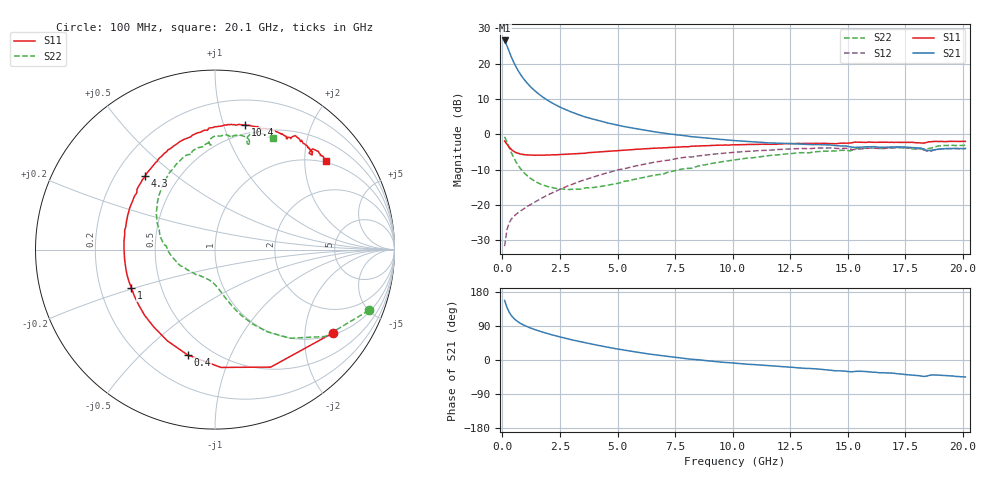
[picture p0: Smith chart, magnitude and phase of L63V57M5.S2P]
!  Infineon Technologies AG
! BFR380L3 , PF131585-7, No.6, Th 09.10.01, soldered on pcb-board, measured with PP GSG850
!  Vce=3.5 V,  Ic=7.5 mA
! Common Emitter S-Parameters:  15. November 2001
#  GHz  S  MA  R  50
! f  S11  S21  S12  S22
! GHz  Mag  Ang  Mag  Ang  Mag  Ang  Mag  Ang
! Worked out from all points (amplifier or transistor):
!   201 points, 100 MHz to 20.1 GHz, reference 50 ohm
!   highest |S21| = 26.5 dB at 100 MHz (marker M1)
!   |S21| within 3 dB of that: start of sweep to 289.7 MHz
!   unconditionally stable (mu >= 1): 1.99 GHz to 4.519 GHz
!   at 3.4 GHz: K = 1.03, MAG = 8.1 dB, |S12| = -13.2 dB
!   at 10.1 GHz: K = 0.94, MSG = 1.6 dB, |S12| = -5.1 dB
!   at 20.1 GHz: K = 0.99, MSG = 0.0 dB, |S12| = -4.0 dB
!   S11 on the Smith chart (normalised r, x): 100 MHz: 1.06, -2.77; 400 MHz: 0.38, -0.70; 1 GHz: 0.34, -0.20; 4.3 GHz: 0.32, +0.39; 10.4 GHz: 0.42, +1.19; 20.1 GHz: 0.95, +2.54
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0.1  0.8036 -35.4  21.17 157.1  0.02627 72.2  0.9217 -21.6
0.2  0.7246 -64.6  17.82 139.0  0.04466 60.2  0.7822 -38.2
0.3  0.6574 -87.1  14.69 126.2  0.05629 52.9  0.6476 -49.7
0.4  0.6068 -104.5  12.21 116.9  0.0638 48.9  0.5422 -57.6
0.5  0.5735 -117.6  10.35 109.9  0.06928 47.2  0.4639 -63.2
0.6  0.5498 -128.3  8.905 104.5  0.07416 46.6  0.4048 -67.4
0.7  0.5368 -136.8  7.816 100.0  0.07855 46.5  0.3594 -70.8
0.8  0.5257 -143.8  6.941 96.3  0.08289 47.0  0.3246 -73.5
1  0.513 -155.2  5.672 90.1  0.09148 48.2  0.2748 -77.8
1.2  0.51 -163.8  4.79 84.9  0.1006 49.7  0.2416 -81.6
1.4  0.5065 -171.1  4.151 80.5  0.11 51.0  0.2186 -84.9
1.6  0.5062 -177.3  3.663 76.3  0.1196 52.2  0.2023 -88.2
1.9  0.5091 174.9  3.125 70.8  0.135 53.3  0.1857 -93.1
2.6  0.5198 160.1  2.344 59.4  0.1725 54.3  0.1688 -105.8
3.5  0.5385 144.7  1.799 46.7  0.224 52.8  0.17 -122.0
4.3  0.565 133.5  1.52 37.0  0.2702 50.1  0.1838 -139.2
6.8  0.6391 104.7  1.062 12.3  0.4145 35.9  0.2702 177.0
10.1  0.7104 78.3  0.8135 -8.4  0.5572 14.1  0.4359 135.5
10.4  0.715 76.3  0.8016 -9.9  0.5676 12.1  0.4487 132.2
13.5  0.7406 60.2  0.716 -22.9  0.6326 -7.8  0.56 103.2
16.8  0.7683 47.6  0.6584 -34.0  0.6373 -24.5  0.6471 79.7
20.1  0.7942 38.7  0.6311 -44.7  0.6289 -38.6  0.7 62.5
